PROGRAM P_Prog6
VAR

	fbKL6401 					: FB_LON_KL6401;

	fbREAD_159		: FB_READ_159_SNVT_pump_sensor;
	fbSEND_159		: FB_SEND_159_SNVT_pump_sensor;

	fbREAD_160		: FB_READ_160_SNVT_abs_humid;
	fbSEND_160		: FB_SEND_160_SNVT_abs_humid;

	fbREAD_161		: FB_READ_161_SNVT_flow_p;
	fbSEND_161		: FB_SEND_161_SNVT_flow_p;

	fbREAD_162		: FB_READ_162_SNVT_dev_c_mode;
	fbSEND_162		: FB_SEND_162_SNVT_dev_c_mode;

	fbREAD_163		: FB_READ_163_SNVT_valve_mode;
	fbSEND_163		: FB_SEND_163_SNVT_valve_mode;

	fbREAD_164		: FB_READ_164_SNVT_alarm_2;
	fbSEND_164		: FB_SEND_164_SNVT_alarm_2;

	fbREAD_165		: FB_READ_165_SNVT_state_64;
	fbSEND_165		: FB_SEND_165_SNVT_state_64;

	fbREAD_166		: FB_READ_166_SNVT_nv_type;
	fbSEND_166		: FB_SEND_166_SNVT_nv_type;
(*
	fbREAD_167		: FB_READ_109_SNVT_occupancy;
	fbSEND_167		: FB_SEND_109_SNVT_occupancy;
*)
	fbREAD_168		: FB_READ_168_SNVT_ent_opmode;
	fbSEND_168		: FB_SEND_168_SNVT_ent_opmode;

	fbREAD_169		: FB_READ_169_SNVT_ent_state;
	fbSEND_169		: FB_SEND_169_SNVT_ent_state;

	fbREAD_170		: FB_READ_170_SNVT_ent_status;
	fbSEND_170		: FB_SEND_170_SNVT_ent_status;

	fbREAD_171		: FB_READ_171_SNVT_flow_dir;
	fbSEND_171		: FB_SEND_171_SNVT_flow_dir;

	fbREAD_172		: FB_READ_172_SNVT_hvac_satsts;
	fbSEND_172		: FB_SEND_172_SNVT_hvac_satsts;

	fbREAD_173		: FB_READ_173_SNVT_dev_status;
	fbSEND_173		: FB_SEND_173_SNVT_dev_status;

	fbREAD_174		: FB_READ_174_SNVT_dev_fault;
	fbSEND_174		: FB_SEND_174_SNVT_dev_fault;

	fbREAD_175		: FB_READ_175_SNVT_dev_maint;
	fbSEND_175		: FB_SEND_175_SNVT_dev_maint;

	fbREAD_176		: FB_READ_176_SNVT_date_event;
	fbSEND_176		: FB_SEND_176_SNVT_date_event;

	fbREAD_177		: FB_READ_177_SNVT_sched_val;
	fbSEND_177		: FB_SEND_177_SNVT_sched_val;

(*
	fbREAD_178		: FB_READ_178;
	fbSEND_178		: FB_SEND_146_SNVT_elec_kwh_l;

	fbREAD_179		: FB_READ_147_SNVT_temp_diff_p;
	fbSEND_179		: FB_SEND_147_SNVT_temp_diff_p;
*)
	fbREAD_180		: FB_READ_180_SNVT_sblnd_state;
	fbSEND_180		: FB_SEND_180_SNVT_sblnd_state;

	fbREAD_181		: FB_READ_181_SNVT_rac_ctrl;
	fbSEND_181		: FB_SEND_181_SNVT_rac_ctrl;

	fbREAD_182		: FB_READ_182_SNVT_rac_req;
	fbSEND_182		: FB_SEND_182_SNVT_rac_req;

	fbREAD_183		: FB_READ_183_SNVT_count_32;
	fbSEND_183		: FB_SEND_183_SNVT_count_32;

	fbREAD_184		: FB_READ_184_SNVT_clothes_w_c;
	fbSEND_184		: FB_SEND_184_SNVT_clothes_w_c;

	fbREAD_185		: FB_READ_185_SNVT_clothes_w_m;
	fbSEND_185		: FB_SEND_185_SNVT_clothes_w_m;

	fbREAD_186		: FB_READ_186_SNVT_clothes_w_s;
	fbSEND_186		: FB_SEND_186_SNVT_clothes_w_s;

	fbREAD_187		: FB_READ_187_SNVT_clothes_w_a;
	fbSEND_187		: FB_SEND_187_SNVT_clothes_w_a;

	fbREAD_188		: FB_READ_188_SNVT_multiplier_s;
	fbSEND_188		: FB_SEND_188_SNVT_multiplier_s;

	fbREAD_189		: FB_READ_189_SNVT_switch_2;
	fbSEND_189		: FB_SEND_189_SNVT_switch_2;

	fbREAD_190		: FB_READ_190_SNVT_color_2;
	fbSEND_190		: FB_SEND_190_SNVT_color_2;

END_VAR


fbKL6401(
	bDisabled:=FALSE ,
	stParameter_IN:=LON_IN_6 ,
	stParameter_OUT:=LON_OUT_6 ,
	stLON_Com:=stLON_Com_6,
	bReady=> ,
	eError=> ,
	stKL6401=> ,
	arrProgID=> ,
	arrNeuronID=> ,
	bBusy=> ,
	bError=> ,
	dwErrorKL=> ,
	bTimeOut=> ,
	byLONState=> );

(**)
fbREAD_159(
	wNVIndex:=0 ,
	bDisabled:= ,
	stLON_Com:=stLON_Com_6,
	stValue=> ,
	bNewData=> ,
	bError=> ,
	eError=> );
fbREAD_159.stValue;
fbREAD_159.bError;
fbREAD_159.eError;

fbSEND_159.stValue;
fbSEND_159.bStart;
fbSEND_159.bError;
fbSEND_159.eError;
fbSEND_159.bBusy;
fbSEND_159.dwErrorKL;

fbSEND_159.bAuto;
fbSEND_159.bSendInit;
fbSEND_159.tMinSendTime;
fbSEND_159.tMaxSendTime;

fbSEND_159(
	wNVIndex:=1 ,
	bStart:= ,
	stValue:= ,
	bDisabled:= ,
	stLON_Com:=stLON_Com_6,
	bError=> ,
	eError=> );
fbSEND_159.bStart:=FALSE;

(**)
fbREAD_160(
	wNVIndex:=2 ,
	bDisabled:= ,
	stLON_Com:=stLON_Com_6,
	rValue=> ,
	bNewData=> ,
	bError=> ,
	eError=> );
fbREAD_160.rValue;
fbREAD_160.bError;
fbREAD_160.eError;

fbSEND_160.rValue;
fbSEND_160.bStart;
fbSEND_160.bError;
fbSEND_160.eError;
fbSEND_160.bBusy;
fbSEND_160.dwErrorKL;

fbSEND_160.bAuto;
fbSEND_160.bSendInit;
fbSEND_160.tMinSendTime;
fbSEND_160.tMaxSendTime;
fbSEND_160.rValueLimit;

fbSEND_160(
	wNVIndex:=3 ,
	bStart:= ,
	rValue:= ,
	bDisabled:= ,
	stLON_Com:=stLON_Com_6,
	bError=> ,
	eError=> );
fbSEND_160.bStart:=FALSE;

(**)
fbREAD_161(
	wNVIndex:=4 ,
	bDisabled:= ,
	stLON_Com:=stLON_Com_6,
	rValue=> ,
	bNewData=> ,
	bError=> ,
	eError=> );
fbREAD_161.rValue;
fbREAD_161.bError;
fbREAD_161.eError;

fbSEND_161.rValue;
fbSEND_161.bStart;
fbSEND_161.bError;
fbSEND_161.eError;
fbSEND_161.bBusy;
fbSEND_161.dwErrorKL;

fbSEND_161.bAuto;
fbSEND_161.bSendInit;
fbSEND_161.tMinSendTime;
fbSEND_161.tMaxSendTime;
fbSEND_161.rValueLimit;

fbSEND_161(
	wNVIndex:=5 ,
	bStart:= ,
	rValue:= ,
	bDisabled:= ,
	stLON_Com:=stLON_Com_6,
	bError=> ,
	eError=> );
fbSEND_161.bStart:=FALSE;

(**)
fbREAD_162(
	wNVIndex:=6 ,
	bDisabled:= ,
	stLON_Com:=stLON_Com_6,
	eValue=> ,
	bNewData=> ,
	bError=> ,
	eError=> );
fbREAD_162.eValue;
fbREAD_162.bError;
fbREAD_162.eError;

fbSEND_162.eValue;
fbSEND_162.bStart;
fbSEND_162.bError;
fbSEND_162.eError;
fbSEND_162.bBusy;
fbSEND_162.dwErrorKL;

fbSEND_162.bAuto;
fbSEND_162.bSendInit;
fbSEND_162.tMinSendTime;
fbSEND_162.tMaxSendTime;

fbSEND_162(
	wNVIndex:=7 ,
	bStart:= ,
	eValue:= ,
	bDisabled:= ,
	stLON_Com:=stLON_Com_6,
	bError=> ,
	eError=> );
fbSEND_162.bStart:=FALSE;

(**)
fbREAD_163(
	wNVIndex:=8 ,
	bDisabled:= ,
	stLON_Com:=stLON_Com_6,
	eValue=> ,
	bNewData=> ,
	bError=> ,
	eError=> );
fbREAD_163.eValue;
fbREAD_163.bError;
fbREAD_163.eError;

fbSEND_163.eValue;
fbSEND_163.bStart;
fbSEND_163.bError;
fbSEND_163.eError;
fbSEND_163.bBusy;
fbSEND_163.dwErrorKL;

fbSEND_163.bAuto;
fbSEND_163.bSendInit;
fbSEND_163.tMinSendTime;
fbSEND_163.tMaxSendTime;

fbSEND_163(
	wNVIndex:=9 ,
	bStart:= ,
	eValue:= ,
	bDisabled:= ,
	stLON_Com:=stLON_Com_6,
	bError=> ,
	eError=> );
fbSEND_163.bStart:=FALSE;

(**)
fbREAD_164(
	wNVIndex:=10 ,
	bDisabled:= ,
	stLON_Com:=stLON_Com_6,
	stValue=> ,
	bNewData=> ,
	bError=> ,
	eError=> );
fbREAD_164.stValue;
fbREAD_164.bError;
fbREAD_164.eError;

fbSEND_164.stValue;
fbSEND_164.bStart;
fbSEND_164.bError;
fbSEND_164.eError;
fbSEND_164.bBusy;
fbSEND_164.dwErrorKL;

fbSEND_164.bAuto;
fbSEND_164.bSendInit;
fbSEND_164.tMinSendTime;
fbSEND_164.tMaxSendTime;

fbSEND_164(
	wNVIndex:=11 ,
	bStart:= ,
	stValue:= ,
	bDisabled:= ,
	stLON_Com:=stLON_Com_6,
	bError=> ,
	eError=> );
fbSEND_164.bStart:=FALSE;

(**)
fbREAD_165(
	wNVIndex:=12 ,
	bDisabled:= ,
	stLON_Com:=stLON_Com_6,
	arrValue=> ,
	bNewData=> ,
	bError=> ,
	eError=> );
fbREAD_165.arrValue;
fbREAD_165.bError;
fbREAD_165.eError;

fbSEND_165.arrValue;
fbSEND_165.bStart;
fbSEND_165.bError;
fbSEND_165.eError;
fbSEND_165.bBusy;
fbSEND_165.dwErrorKL;

fbSEND_165.bAuto;
fbSEND_165.bSendInit;
fbSEND_165.tMinSendTime;
fbSEND_165.tMaxSendTime;

fbSEND_165(
	wNVIndex:=13 ,
	bStart:= ,
	arrValue:= ,
	bDisabled:= ,
	stLON_Com:=stLON_Com_6,
	bError=> ,
	eError=> );
fbSEND_165.bStart:=FALSE;

(**)
fbREAD_166(
	wNVIndex:=14 ,
	bDisabled:= ,
	stLON_Com:=stLON_Com_6,
	stValue=> ,
	bNewData=> ,
	bError=> ,
	eError=> );
fbREAD_166.stValue;
fbREAD_166.bError;
fbREAD_166.eError;

(*fbSEND_166.stValue.arrType_program_ID:=P_Prog0.fbKL6401.arrProgID;*)
fbSEND_166.stValue;
fbSEND_166.bStart;
fbSEND_166.bError;
fbSEND_166.eError;
fbSEND_166.bBusy;
fbSEND_166.dwErrorKL;

fbSEND_166.bAuto;
fbSEND_166.bSendInit;
fbSEND_166.tMinSendTime;
fbSEND_166.tMaxSendTime;

fbSEND_166(
	wNVIndex:=15 ,
	bStart:= ,
	stValue:= ,
	bDisabled:= ,
	stLON_Com:=stLON_Com_6,
	bError=> ,
	eError=> );
fbSEND_166.bStart:=FALSE;

(*67*)

(**)
fbREAD_168(
	wNVIndex:=16 ,
	bDisabled:= ,
	stLON_Com:=stLON_Com_6,
	eValue=> ,
	bNewData=> ,
	bError=> ,
	eError=> );
fbREAD_168.eValue;
fbREAD_168.bError;
fbREAD_168.eError;

fbSEND_168.eValue;
fbSEND_168.bStart;
fbSEND_168.bError;
fbSEND_168.eError;
fbSEND_168.bBusy;
fbSEND_168.dwErrorKL;

fbSEND_168.bAuto;
fbSEND_168.bSendInit;
fbSEND_168.tMinSendTime;
fbSEND_168.tMaxSendTime;

fbSEND_168(
	wNVIndex:=17 ,
	bStart:= ,
	eValue:= ,
	bDisabled:= ,
	stLON_Com:=stLON_Com_6,
	bError=> ,
	eError=> );
fbSEND_168.bStart:=FALSE;

(**)
fbREAD_169(
	wNVIndex:=18 ,
	bDisabled:= ,
	stLON_Com:=stLON_Com_6,
	eValue=> ,
	bNewData=> ,
	bError=> ,
	eError=> );
fbREAD_169.eValue;
fbREAD_169.bError;
fbREAD_169.eError;

fbSEND_169.eValue;
fbSEND_169.bStart;
fbSEND_169.bError;
fbSEND_169.eError;
fbSEND_169.bBusy;
fbSEND_169.dwErrorKL;

fbSEND_169.bAuto;
fbSEND_169.bSendInit;
fbSEND_169.tMinSendTime;
fbSEND_169.tMaxSendTime;

fbSEND_169(
	wNVIndex:=19 ,
	bStart:= ,
	eValue:= ,
	bDisabled:= ,
	stLON_Com:=stLON_Com_6,
	bError=> ,
	eError=> );
fbSEND_169.bStart:=FALSE;

(**)
fbREAD_170(
	wNVIndex:=20 ,
	bDisabled:= ,
	stLON_Com:=stLON_Com_6,
	stValue=> ,
	bNewData=> ,
	bError=> ,
	eError=> );
fbREAD_170.stValue;
fbREAD_170.bError;
fbREAD_170.eError;

fbSEND_170.stValue;
fbSEND_170.bStart;
fbSEND_170.bError;
fbSEND_170.eError;
fbSEND_170.bBusy;
fbSEND_170.dwErrorKL;

fbSEND_170.bAuto;
fbSEND_170.bSendInit;
fbSEND_170.tMinSendTime;
fbSEND_170.tMaxSendTime;

fbSEND_170(
	wNVIndex:=21 ,
	bStart:= ,
	stValue:= ,
	bDisabled:= ,
	stLON_Com:=stLON_Com_6,
	bError=> ,
	eError=> );
fbSEND_170.bStart:=FALSE;

(**)
fbREAD_171(
	wNVIndex:=22 ,
	bDisabled:= ,
	stLON_Com:=stLON_Com_6,
	eValue=> ,
	bNewData=> ,
	bError=> ,
	eError=> );
fbREAD_171.eValue;
fbREAD_171.bError;
fbREAD_171.eError;

fbSEND_171.eValue;
fbSEND_171.bStart;
fbSEND_171.bError;
fbSEND_171.eError;
fbSEND_171.bBusy;
fbSEND_171.dwErrorKL;

fbSEND_171.bAuto;
fbSEND_171.bSendInit;
fbSEND_171.tMinSendTime;
fbSEND_171.tMaxSendTime;

fbSEND_171(
	wNVIndex:=23 ,
	bStart:= ,
	eValue:= ,
	bDisabled:= ,
	stLON_Com:=stLON_Com_6,
	bError=> ,
	eError=> );
fbSEND_171.bStart:=FALSE;

(**)
fbREAD_172(
	wNVIndex:=24 ,
	bDisabled:= ,
	stLON_Com:=stLON_Com_6,
	stValue=> ,
	bNewData=> ,
	bError=> ,
	eError=> );
fbREAD_172.stValue;
fbREAD_172.bError;
fbREAD_172.eError;

fbSEND_172.stValue;
fbSEND_172.bStart;
fbSEND_172.bError;
fbSEND_172.eError;
fbSEND_172.bBusy;
fbSEND_172.dwErrorKL;

fbSEND_172.bAuto;
fbSEND_172.bSendInit;
fbSEND_172.tMinSendTime;
fbSEND_172.tMaxSendTime;

fbSEND_172(
	wNVIndex:=25 ,
	bStart:= ,
	stValue:= ,
	bDisabled:= ,
	stLON_Com:=stLON_Com_6,
	bError=> ,
	eError=> );
fbSEND_172.bStart:=FALSE;

(**)
fbREAD_173(
	wNVIndex:=26 ,
	bDisabled:= ,
	stLON_Com:=stLON_Com_6,
	stValue=> ,
	bNewData=> ,
	bError=> ,
	eError=> );
fbREAD_173.stValue;
fbREAD_173.bError;
fbREAD_173.eError;

fbSEND_173.stValue;
fbSEND_173.bStart;
fbSEND_173.bError;
fbSEND_173.eError;
fbSEND_173.bBusy;
fbSEND_173.dwErrorKL;

fbSEND_173.bAuto;
fbSEND_173.bSendInit;
fbSEND_173.tMinSendTime;
fbSEND_173.tMaxSendTime;

fbSEND_173(
	wNVIndex:=27 ,
	bStart:= ,
	stValue:= ,
	bDisabled:= ,
	stLON_Com:=stLON_Com_6,
	bError=> ,
	eError=> );
fbSEND_173.bStart:=FALSE;

(**)
fbREAD_174(
	wNVIndex:=28 ,
	bDisabled:= ,
	stLON_Com:=stLON_Com_6,
	stValue=> ,
	bNewData=> ,
	bError=> ,
	eError=> );
fbREAD_174.stValue;
fbREAD_174.bError;
fbREAD_174.eError;

fbSEND_174.stValue;
fbSEND_174.bStart;
fbSEND_174.bError;
fbSEND_174.eError;
fbSEND_174.bBusy;
fbSEND_174.dwErrorKL;

fbSEND_174.bAuto;
fbSEND_174.bSendInit;
fbSEND_174.tMinSendTime;
fbSEND_174.tMaxSendTime;

fbSEND_174(
	wNVIndex:=29 ,
	bStart:= ,
	stValue:= ,
	bDisabled:= ,
	stLON_Com:=stLON_Com_6,
	bError=> ,
	eError=> );
fbSEND_174.bStart:=FALSE;

(**)
fbREAD_175(
	wNVIndex:=30 ,
	bDisabled:= ,
	stLON_Com:=stLON_Com_6,
	stValue=> ,
	bNewData=> ,
	bError=> ,
	eError=> );
fbREAD_175.stValue;
fbREAD_175.bError;
fbREAD_175.eError;

fbSEND_175.stValue;
fbSEND_175.bStart;
fbSEND_175.bError;
fbSEND_175.eError;
fbSEND_175.bBusy;
fbSEND_175.dwErrorKL;

fbSEND_175.bAuto;
fbSEND_175.bSendInit;
fbSEND_175.tMinSendTime;
fbSEND_175.tMaxSendTime;

fbSEND_175(
	wNVIndex:=31 ,
	bStart:= ,
	stValue:= ,
	bDisabled:= ,
	stLON_Com:=stLON_Com_6,
	bError=> ,
	eError=> );
fbSEND_175.bStart:=FALSE;

(**)
fbREAD_176(
	wNVIndex:=32 ,
	bDisabled:= ,
	stLON_Com:=stLON_Com_6,
	stValue=> ,
	bNewData=> ,
	bError=> ,
	eError=> );
fbREAD_176.stValue;
fbREAD_176.bError;
fbREAD_176.eError;

fbSEND_176.stValue;
fbSEND_176.bStart;
fbSEND_176.bError;
fbSEND_176.eError;
fbSEND_176.bBusy;
fbSEND_176.dwErrorKL;

fbSEND_176.bAuto;
fbSEND_176.bSendInit;
fbSEND_176.tMinSendTime;
fbSEND_176.tMaxSendTime;

fbSEND_176(
	wNVIndex:=33 ,
	bStart:= ,
	stValue:= ,
	bDisabled:= ,
	stLON_Com:=stLON_Com_6,
	bError=> ,
	eError=> );
fbSEND_176.bStart:=FALSE;

(**)
fbREAD_177(
	wNVIndex:=34 ,
	bDisabled:= ,
	stLON_Com:=stLON_Com_6,
	byValue=> ,
	bNewData=> ,
	bError=> ,
	eError=> );
fbREAD_177.byValue;
fbREAD_177.bError;
fbREAD_177.eError;

fbSEND_177.byValue;
fbSEND_177.bStart;
fbSEND_177.bError;
fbSEND_177.eError;
fbSEND_177.bBusy;
fbSEND_177.dwErrorKL;

fbSEND_177.bAuto;
fbSEND_177.bSendInit;
fbSEND_177.tMinSendTime;
fbSEND_177.tMaxSendTime;
fbSEND_177.byValueLimit;

fbSEND_177(
	wNVIndex:=35 ,
	bStart:= ,
	byValue:= ,
	bDisabled:= ,
	stLON_Com:=stLON_Com_6,
	bError=> ,
	eError=> );
fbSEND_177.bStart:=FALSE;

(*78 /36 / 37*)
(*79 /38 / 39*)

(**)
fbREAD_180(
	wNVIndex:=40 ,
	bDisabled:= ,
	stLON_Com:=stLON_Com_6,
	stValue=> ,
	bNewData=> ,
	bError=> ,
	eError=> );
fbREAD_180.stValue;
fbREAD_180.bError;
fbREAD_180.eError;

fbSEND_180.stValue;
fbSEND_180.bStart;
fbSEND_180.bError;
fbSEND_180.eError;
fbSEND_180.bBusy;
fbSEND_180.dwErrorKL;

fbSEND_180.bAuto;
fbSEND_180.bSendInit;
fbSEND_180.tMinSendTime;
fbSEND_180.tMaxSendTime;

fbSEND_180(
	wNVIndex:=41 ,
	bStart:= ,
	stValue:= ,
	bDisabled:= ,
	stLON_Com:=stLON_Com_6,
	bError=> ,
	eError=> );
fbSEND_180.bStart:=FALSE;

(**)
fbREAD_181(
	wNVIndex:=42 ,
	bDisabled:= ,
	stLON_Com:=stLON_Com_6,
	stValue=> ,
	bNewData=> ,
	bError=> ,
	eError=> );
fbREAD_181.stValue;
fbREAD_181.bError;
fbREAD_181.eError;

fbSEND_181.stValue;
fbSEND_181.bStart;
fbSEND_181.bError;
fbSEND_181.eError;
fbSEND_181.bBusy;
fbSEND_181.dwErrorKL;

fbSEND_181.bAuto;
fbSEND_181.bSendInit;
fbSEND_181.tMinSendTime;
fbSEND_181.tMaxSendTime;

fbSEND_181(
	wNVIndex:=43 ,
	bStart:= ,
	stValue:= ,
	bDisabled:= ,
	stLON_Com:=stLON_Com_6,
	bError=> ,
	eError=> );
fbSEND_181.bStart:=FALSE;

(**)
fbREAD_182(
	wNVIndex:=44 ,
	bDisabled:= ,
	stLON_Com:=stLON_Com_6,
	stValue=> ,
	bNewData=> ,
	bError=> ,
	eError=> );
fbREAD_182.stValue;
fbREAD_182.bError;
fbREAD_182.eError;

fbSEND_182.stValue;
fbSEND_182.bStart;
fbSEND_182.bError;
fbSEND_182.eError;
fbSEND_182.bBusy;
fbSEND_182.dwErrorKL;

fbSEND_182.bAuto;
fbSEND_182.bSendInit;
fbSEND_182.tMinSendTime;
fbSEND_182.tMaxSendTime;

fbSEND_182(
	wNVIndex:=45 ,
	bStart:= ,
	stValue:= ,
	bDisabled:= ,
	stLON_Com:=stLON_Com_6,
	bError=> ,
	eError=> );
fbSEND_182.bStart:=FALSE;

(**)
fbREAD_183(
	wNVIndex:=46 ,
	bDisabled:= ,
	stLON_Com:=stLON_Com_6,
	udiValue=> ,
	bNewData=> ,
	bError=> ,
	eError=> );
fbREAD_183.udiValue;
fbREAD_183.bError;
fbREAD_183.eError;

fbSEND_183.udiValue;
fbSEND_183.bStart;
fbSEND_183.bError;
fbSEND_183.eError;
fbSEND_183.bBusy;
fbSEND_183.dwErrorKL;

fbSEND_183.bAuto;
fbSEND_183.bSendInit;
fbSEND_183.tMinSendTime;
fbSEND_183.tMaxSendTime;
fbSEND_183.udiValueLimit;

fbSEND_183(
	wNVIndex:=47 ,
	bStart:= ,
	udiValue:= ,
	bDisabled:= ,
	stLON_Com:=stLON_Com_6,
	bError=> ,
	eError=> );
fbSEND_183.bStart:=FALSE;

(**)
fbREAD_184(
	wNVIndex:=48 ,
	bDisabled:= ,
	stLON_Com:=stLON_Com_6,
	stValue=> ,
	bNewData=> ,
	bError=> ,
	eError=> );
fbREAD_184.stValue;
fbREAD_184.bError;
fbREAD_184.eError;

fbREAD_184.stValue.eCycle;
fbREAD_184.stValue.eCycle;
fbREAD_184.stValue.byRervd;

fbREAD_184.stValue.stAction.bPower_on;
fbREAD_184.stValue.stAction.bRun_mode;
fbREAD_184.stValue.stAction.byRsrvd2_7;

fbREAD_184.stValue.stFunction.eProgram;
fbREAD_184.stValue.stFunction.stWash.eLoad_level;
fbREAD_184.stValue.stFunction.stWash.byTemp;
fbREAD_184.stValue.stFunction.stWash.byTime;
fbREAD_184.stValue.stFunction.stWash.ePrewash;

fbREAD_184.stValue.stFunction.stRinse.byTemp;
fbREAD_184.stValue.stFunction.stRinse.byRepeat;
fbREAD_184.stValue.stFunction.stRinse.eOption;

fbREAD_184.stValue.stFunction.stSpin.uiSpeed;
fbREAD_184.stValue.stFunction.stSpin.byTime;
fbREAD_184.stValue.stFunction.stSpin.eHold;

fbREAD_184.stValue.stFunction.stDry.byTemp;
fbREAD_184.stValue.stFunction.stDry.stDuration.byTime;
fbREAD_184.stValue.stFunction.stDry.stDuration.eDryness;

fbREAD_184.stValue.uiTime_remaining;

fbSEND_184.stValue;
fbSEND_184.bStart;
fbSEND_184.bError;
fbSEND_184.eError;
fbSEND_184.bBusy;
fbSEND_184.dwErrorKL;

fbSEND_184.bAuto;
fbSEND_184.bSendInit;
fbSEND_184.tMinSendTime;
fbSEND_184.tMaxSendTime;

fbSEND_184.stValue.eCycle;
fbSEND_184.stValue.eCycle;
fbSEND_184.stValue.byRervd;

fbSEND_184.stValue.stAction.bPower_on;
fbSEND_184.stValue.stAction.bRun_mode;
fbSEND_184.stValue.stAction.byRsrvd2_7;

fbSEND_184.stValue.stFunction.eProgram;
fbSEND_184.stValue.stFunction.stWash.eLoad_level;
fbSEND_184.stValue.stFunction.stWash.byTemp;
fbSEND_184.stValue.stFunction.stWash.byTime;
fbSEND_184.stValue.stFunction.stWash.ePrewash;

fbSEND_184.stValue.stFunction.stRinse.byTemp;
fbSEND_184.stValue.stFunction.stRinse.byRepeat;
fbSEND_184.stValue.stFunction.stRinse.eOption;

fbSEND_184.stValue.stFunction.stSpin.uiSpeed;
fbSEND_184.stValue.stFunction.stSpin.byTime;
fbSEND_184.stValue.stFunction.stSpin.eHold;

fbSEND_184.stValue.stFunction.stDry.byTemp;
fbSEND_184.stValue.stFunction.stDry.stDuration.byTime;
fbSEND_184.stValue.stFunction.stDry.stDuration.eDryness;

fbSEND_184.stValue.uiTime_remaining;

fbSEND_184(
	wNVIndex:=49 ,
	bStart:= ,
	stValue:= ,
	bDisabled:= ,
	stLON_Com:=stLON_Com_6,
	bError=> ,
	eError=> );
fbSEND_184.bStart:=FALSE;

(**)
fbREAD_185(
	wNVIndex:=50 ,
	bDisabled:= ,
	stLON_Com:=stLON_Com_6,
	stValue=> ,
	bNewData=> ,
	bError=> ,
	eError=> );
fbREAD_185.stValue;
fbREAD_185.bError;
fbREAD_185.eError;

fbSEND_185.stValue;
fbSEND_185.bStart;
fbSEND_185.bError;
fbSEND_185.eError;
fbSEND_185.bBusy;
fbSEND_185.dwErrorKL;

fbSEND_185.bAuto;
fbSEND_185.bSendInit;
fbSEND_185.tMinSendTime;
fbSEND_185.tMaxSendTime;

fbSEND_185(
	wNVIndex:=51 ,
	bStart:= ,
	stValue:= ,
	bDisabled:= ,
	stLON_Com:=stLON_Com_6,
	bError=> ,
	eError=> );
fbSEND_185.bStart:=FALSE;

(**)
fbREAD_186(
	wNVIndex:=52 ,
	bDisabled:= ,
	stLON_Com:=stLON_Com_6,
	stValue=> ,
	bNewData=> ,
	bError=> ,
	eError=> );
fbREAD_186.stValue;
fbREAD_186.bError;
fbREAD_186.eError;

fbSEND_186.stValue;
fbSEND_186.bStart;
fbSEND_186.bError;
fbSEND_186.eError;
fbSEND_186.bBusy;
fbSEND_186.dwErrorKL;

fbSEND_186.bAuto;
fbSEND_186.bSendInit;
fbSEND_186.tMinSendTime;
fbSEND_186.tMaxSendTime;

fbSEND_186(
	wNVIndex:=53 ,
	bStart:= ,
	stValue:= ,
	bDisabled:= ,
	stLON_Com:=stLON_Com_6,
	bError=> ,
	eError=> );
fbSEND_186.bStart:=FALSE;

(**)
fbREAD_187(
	wNVIndex:=54 ,
	bDisabled:= ,
	stLON_Com:=stLON_Com_6,
	stValue=> ,
	bNewData=> ,
	bError=> ,
	eError=> );
fbREAD_187.stValue;
fbREAD_187.bError;
fbREAD_187.eError;

fbSEND_187.stValue;
fbSEND_187.bStart;
fbSEND_187.bError;
fbSEND_187.eError;
fbSEND_187.bBusy;
fbSEND_187.dwErrorKL;

fbSEND_187.bAuto;
fbSEND_187.bSendInit;
fbSEND_187.tMinSendTime;
fbSEND_187.tMaxSendTime;

fbSEND_187(
	wNVIndex:=55 ,
	bStart:= ,
	stValue:= ,
	bDisabled:= ,
	stLON_Com:=stLON_Com_6,
	bError=> ,
	eError=> );
fbSEND_187.bStart:=FALSE;

(**)
fbREAD_188(
	wNVIndex:=56 ,
	bDisabled:= ,
	stLON_Com:=stLON_Com_6,
	rValue=> ,
	bNewData=> ,
	bError=> ,
	eError=> );
fbREAD_188.rValue;
fbREAD_188.bError;
fbREAD_188.eError;

fbSEND_188.rValue;
fbSEND_188.bStart;
fbSEND_188.bError;
fbSEND_188.eError;
fbSEND_188.bBusy;
fbSEND_188.dwErrorKL;

fbSEND_188.bAuto;
fbSEND_188.bSendInit;
fbSEND_188.tMinSendTime;
fbSEND_188.tMaxSendTime;
fbSEND_188.rValueLimit;

fbSEND_188(
	wNVIndex:=57 ,
	bStart:= ,
	rValue:= ,
	bDisabled:= ,
	stLON_Com:=stLON_Com_6,
	bError=> ,
	eError=> );
fbSEND_188.bStart:=FALSE;

(**)
fbREAD_189(
	wNVIndex:=58 ,
	bDisabled:= ,
	stLON_Com:=stLON_Com_6,
	stValue=> ,
	bNewData=> ,
	bError=> ,
	eError=> );
fbREAD_189.stValue;
fbREAD_189.bError;
fbREAD_189.eError;

fbSEND_189.stValue;
fbSEND_189.bStart;
fbSEND_189.bError;
fbSEND_189.eError;
fbSEND_189.bBusy;
fbSEND_189.dwErrorKL;

fbSEND_189.bAuto;
fbSEND_189.bSendInit;
fbSEND_189.tMinSendTime;
fbSEND_189.tMaxSendTime;

fbSEND_189(
	wNVIndex:=59 ,
	bStart:= ,
	stValue:= ,
	bDisabled:= ,
	stLON_Com:=stLON_Com_6,
	bError=> ,
	eError=> );
fbSEND_189.bStart:=FALSE;

(**)
fbREAD_190(
	wNVIndex:=60 ,
	bDisabled:= ,
	stLON_Com:=stLON_Com_6,
	stValue=> ,
	bNewData=> ,
	bError=> ,
	eError=> );
fbREAD_190.stValue;
fbREAD_190.bError;
fbREAD_190.eError;

fbSEND_190.stValue;
fbSEND_190.bStart;
fbSEND_190.bError;
fbSEND_190.eError;
fbSEND_190.bBusy;
fbSEND_190.dwErrorKL;

fbSEND_190.bAuto;
fbSEND_190.bSendInit;
fbSEND_190.tMinSendTime;
fbSEND_190.tMaxSendTime;

fbSEND_190(
	wNVIndex:=61 ,
	bStart:= ,
	stValue:= ,
	bDisabled:= ,
	stLON_Com:=stLON_Com_6,
	bError=> ,
	eError=> );
fbSEND_190.bStart:=FALSE;

END_PROGRAM
